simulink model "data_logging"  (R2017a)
settings: Solver=ode45  StartTime=0.0  StopTime=0.1  RelTol=1e-3  EnableMultiTasking=on
InitFcn:
  | Ts_box = 10e-6;
  | Ns_datacap = 50;
  | Ts_udp = 10e-3;
undefined symbols (not defined in the file or in its folder): plecs

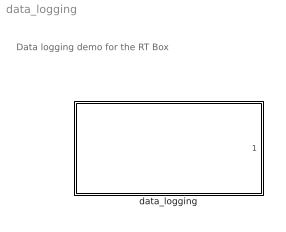
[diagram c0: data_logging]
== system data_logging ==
  note: Data logging demo for the RT Box
  data_logging : Subsystem  LoadFcn=plecs('sl', 200);  InitFcn=plecs('sl', 214);  StartFcn=plecs('sl', 208);  StopFcn=plecs('sl', 209);  ClipboardFcn=plecs('sl', 212, 2);

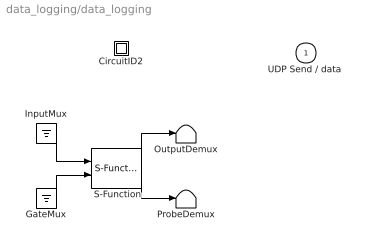
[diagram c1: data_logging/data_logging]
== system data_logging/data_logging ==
  " CircuitID2 " : Subsystem
  " GateMux " : Ground
  " InputMux " : Ground
  " OutputDemux " : Terminator
  " ProbeDemux " : Terminator
  " S-Function " : S-Function  FunctionName=plecs  SFunctionDeploymentMode=off  EnableBusSupport=off
  "UDP Send / data " : Outport  PortDimensions=1
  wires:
  " InputMux "/1 -> " S-Function "/1
  " GateMux "/1 -> " S-Function "/2
  " S-Function "/1 -> " OutputDemux "/1
  " S-Function "/2 -> " ProbeDemux "/1

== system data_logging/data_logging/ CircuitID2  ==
